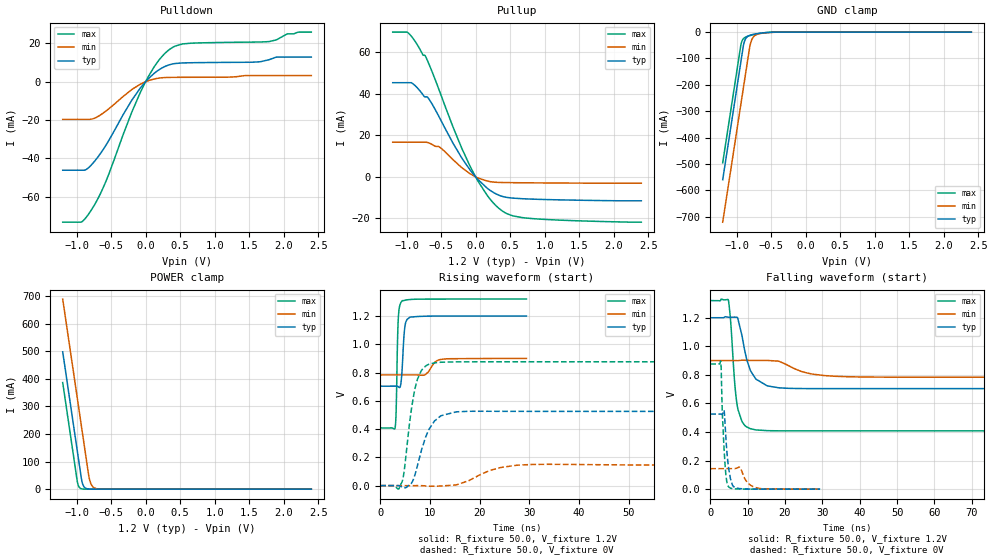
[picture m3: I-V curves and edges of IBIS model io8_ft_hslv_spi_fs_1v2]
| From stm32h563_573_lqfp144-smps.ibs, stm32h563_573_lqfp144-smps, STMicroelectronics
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[Model]   io8_ft_hslv_spi_fs_1v2
Model_type I/O
Polarity   Non-Inverting
Enable   Active-Low
| CAP_THRESHOLD on pad IOFT is "UDTCAPC" :
| Rising=20.0% of vddiom   Falling=80.0% of vddiom
| C_comp min and max val. don't necessarily correlate with the min and max pvt
| but are the smallest and greatest pad capacitance found.
| var   typ   min   max
C_comp   4.03040pF  3.93195pF  4.03605pF
|C_comp_pullup   2.46595pF  2.28040pF  2.18970pF
|C_comp_pulldown   1.56445pF  1.65155pF  1.84635pF
Vinl = 270.0mV
Vinh = 924.0mV
Vmeas = 600.0mV   | Reference voltage for timing measurements
Cref  = 50.0pF   | Timing specification test load capacitance value
Rref  = 100.0MOhm   | Timing specification test load resistance value
Vref  = 600.0mV   | Timing specification test load voltage
[Model Spec]
| TIME_THRESHOLD on pin ZIV11 is "CMOS" :
| Rising=40.0% of vdd   Falling=60.0% of vdd
Vinl 447.80000mV 344.80000mV 489.80000mV
Vinh 733.20000mV 535.20000mV 813.20000mV
| variable   typ   min   max
[Temperature Range] 25.0 125.0 -40.0
| variable   typ   min   max
[Voltage Range] 1.2V 900.0mV 1.32V
| variable   typ   min   max
[POWER Clamp Reference] 1.2V 900.0mV 1.32V
| variable   typ   min   max
[GND Clamp Reference] 0V 0V 0V
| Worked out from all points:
|   slope of the pulldown table from 0 to 0.18 V, typ, clamps not added: 30.6 ohm
|   slope of the pullup table from 0 to 0.18 V, typ, clamps not added: 31.3 ohm
|   GND clamp passes 1 mA (typ) near -0.52 V on its own axis
|   POWER clamp passes 1 mA (typ) near -0.84 V on its own axis
|   rising waveform, R_fixture 50.0, V_fixture 1.2V: 20-80 % time 514ps typ, 1.42ns min, 331ps max; typ from 0.704 V to 1.2 V
|   falling waveform, R_fixture 50.0, V_fixture 1.2V: 20-80 % time 3.16ns typ, 7.09ns min, 1.63ns max; typ from 1.2 V to 0.704 V
|   rising waveform, R_fixture 50.0, V_fixture 0V: 20-80 % time 3.01ns typ, 5.55ns min, 2.03ns max; typ from 0 V to 0.525 V
|   falling waveform, R_fixture 50.0, V_fixture 0V: 20-80 % time 1.15ns typ, 2.13ns min, 895ps max; typ from 0.525 V to 0 V
[POWER Clamp]
-1.2V     497.8mA    689.2mA    386.5mA
-990mV    140.8mA    332.2mA    29.53mA
-980mV    123.8mA    315.2mA    17.95mA
-960mV    89.81mA    281.2mA    6.634mA
-930mV    38.81mA    230.2mA    1.49mA
-900mV    12.07mA    179.2mA    334.8uA
-870mV    3.756mA    128.2mA    75.22uA
-820mV    536.4uA    44.98mA    6.246uA
-790mV    166.9uA    18.76mA    1.403uA
-750mV    35.18uA    5.846mA    191.9nA
-590mV    70.47nA    54.99uA    202.5pA
2.4V      0A         0A         0A
[GND Clamp]
-1.2V     -559.6mA   -720.6mA   -495.5mA
-940mV    -117.6mA   -278.6mA   -53.46mA
-930mV    -100.6mA   -261.6mA   -41.27mA
-900mV    -50.49mA   -210.6mA   -24.86mA
-880mV    -31.4mA    -176.6mA   -20.57mA
-850mV    -18.9mA    -125.6mA   -16.88mA
-810mV    -12.57mA   -58.3mA    -13.49mA
-780mV    -10.11mA   -29.57mA   -11.38mA
-740mV    -7.754mA   -14.31mA   -8.91mA
-640mV    -3.713mA   -4.821mA   -4.078mA
-390mV    -82.2uA    -288.6uA   -29.73uA
2.4V      3.859nA    727.3nA    172.3pA
| variable   typ   min   max
[Pullup Reference] 1.2V 900.0mV 1.32V
| variable   typ   min   max
[Pulldown Reference] 0V 0V 0V
[Pullup]
-1.2V     45.24mA    16.65mA    69.55mA
-990mV    45.24mA    16.65mA    69.55mA
-900mV    44.53mA    16.65mA    66.26mA
-730mV    38.43mA    16.65mA    58.24mA
-680mV    37.61mA    16.35mA    54.55mA
-510mV    27.67mA    13.99mA    40.11mA
-80mV     3.3mA      1.496mA    5.118mA
170mV     -5.495mA   -2.025mA   -8.99mA
360mV     -9.094mA   -2.702mA   -15.73mA
540mV     -10.23mA   -2.8mA     -18.76mA
790mV     -10.67mA   -2.88mA    -19.97mA
2.4V      -11.52mA   -3.045mA   -21.79mA
[Pulldown]
-1.2V     -46.17mA   -19.62mA   -73.27mA
-930mV    -46.17mA   -19.62mA   -73.17mA
-770mV    -42.8mA    -19.41mA   -66.04mA
-570mV    -32.88mA   -15.18mA   -51.58mA
-200mV    -9.658mA   -4.084mA   -15.89mA
-80mV     -3.488mA   -1.363mA   -5.887mA
140mV     4.817mA    1.546mA    8.585mA
340mV     8.782mA    2.251mA    16.66mA
540mV     9.805mA    2.305mA    19.74mA
1.79V     11.49mA    3.197mA    20.93mA
2.05V     12.83mA    3.197mA    24.95mA
2.4V      12.83mA    3.197mA    25.89mA
[Ramp]
dV/dt_r 315.17761mV/2.93951ns 86.14942mV/5.33663ns 525.78542mV/2.0277ns
dV/dt_f 297.79714mV/3.0056ns 69.9229mV/7.01152ns 547.13923mV/1.62831ns
R_load = 50.0
| Removed startup time: 0s 0s 0s  .
| Removed end time: 29.4ns.
[Rising Waveform]
R_fixture   = 50.0
V_fixture   = 1.2V
V_fixture_min = 900.0mV
V_fixture_max = 1.32V
0s        703.7mV    783.5mV    408.1mV
3ns       704mV      783.4mV    412.5mV
3.2ns     704.2mV    783.5mV    538.8mV
3.6ns     700.1mV    783.5mV    1.167V
4.05ns    704.3mV    783.5mV    1.287V
4.4ns     826.7mV    783.5mV    1.307V
5ns       1.136V     783.5mV    1.312V
6ns       1.192V     783.5mV    1.317V
12.6ns    1.2V       895mV      1.32V
29.4ns    1.2V       899.9mV    1.32V
| Removed startup time: 0s 0s 0s  .
| Removed end time: 149.4ns.
[Falling Waveform]
R_fixture   = 50.0
V_fixture   = 1.2V
V_fixture_min = 900.0mV
V_fixture_max = 1.32V
0s        1.2V       900mV      1.32V
4.85ns    1.203V     900mV      1.322V
5.5ns     1.203V     900mV      1.157V
6.55ns    1.204V     899.9mV    740.5mV
7.25ns    1.201V     899.6mV    579.9mV
8.55ns    1.065V     902.7mV    470.8mV
10.75ns   830mV      901mV      423.1mV
20.35ns   706.4mV    872.6mV    408.2mV
36.6ns    703.7mV    787.1mV    408.1mV
149.4ns   703.7mV    783.5mV    408.1mV
| Removed startup time: 0s 0s 0s  .
| Removed end time: 149.4ns.
[Rising Waveform]
R_fixture   = 50.0
V_fixture   = 0V
V_fixture_min = 0V
V_fixture_max = 0V
0s        166.4nV    850.9nV    114.3nV
4.3ns     -8.355mV   -526.4nV   20.33mV
4.8ns     -13.15mV   460.8nV    102.1mV
6.2ns     14.35mV    -10uV      524.4mV
7.3ns     118mV      108.1uV    731.7mV
9.1ns     340.9mV    -2.152mV   845.9mV
10.9ns    457.3mV    -4.302mV   868.5mV
15.3ns    522.3mV    5.208mV    875.6mV
30.5ns    525.4mV    149.7mV    876.2mV
149.4ns   525.3mV    143.6mV    876.3mV
| Removed startup time: 0s 0s 0s  .
| Removed end time: 29.4ns.
[Falling Waveform]
R_fixture   = 50.0
V_fixture   = 0V
V_fixture_min = 0V
V_fixture_max = 0V
0s        525.3mV    143.6mV    876.3mV
2.8ns     525.4mV    143.6mV    897mV
2.9ns     525.3mV    143.6mV    856.9mV
3.25ns    527.1mV    143.6mV    515.7mV
3.85ns    505.3mV    143.6mV    212.4mV
4.35ns    295.1mV    143.6mV    63.41mV
4.95ns    140.4mV    143.6mV    15.02mV
6.6ns     9.875mV    143.9mV    2.059mV
12.6ns    441.6uV    8.152mV    147.8uV
29.4ns    2.656uV    129.5uV    422.2nV
